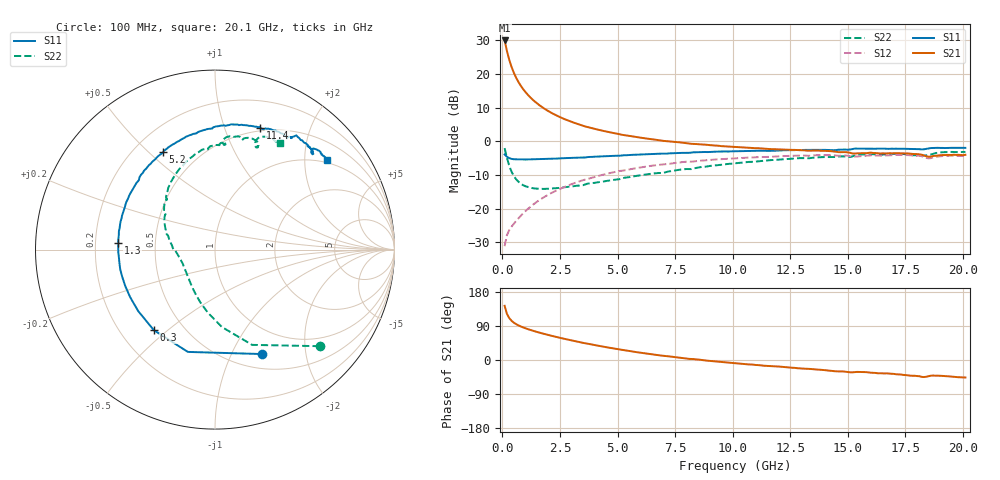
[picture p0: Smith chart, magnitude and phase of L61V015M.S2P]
!  Infineon Technologies AG
! BFR380L3 , PF131585-7, No.6, Th 09.10.01, soldered on pcb-board, measured with PP GSG850
!  Vce=1.0 V,  Ic=15.0 mA
! Common Emitter S-Parameters:  15. November 2001
#  GHz  S  MA  R  50
! f  S11  S21  S12  S22
! GHz  Mag  Ang  Mag  Ang  Mag  Ang  Mag  Ang
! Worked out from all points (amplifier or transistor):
!   201 points, 100 MHz to 20.1 GHz, reference 50 ohm
!   highest |S21| = 30.0 dB at 100 MHz (marker M1)
!   |S21| within 3 dB of that: start of sweep to 197.3 MHz
!   unconditionally stable (mu >= 1): 1.468 GHz to 4.926 GHz
!   at 3.4 GHz: K = 1.03, MAG = 7.3 dB, |S12| = -11.8 dB
!   at 10.1 GHz: K = 0.97, MSG = 1.7 dB, |S12| = -5.1 dB
!   at 20.1 GHz: K = 0.99, MSG = 0.1 dB, |S12| = -4.3 dB
!   S11 on the Smith chart (normalised r, x): 100 MHz: 0.67, -1.32; 300 MHz: 0.34, -0.45; 1.3 GHz: 0.30, +0.03; 5.2 GHz: 0.32, +0.56; 11.4 GHz: 0.47, +1.33; 20.1 GHz: 0.93, +2.56
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0.1  0.639 -65.6  31.62 142.9  0.02762 61.6  0.7934 -42.7
0.2  0.5897 -104.9  22.17 122.0  0.04024 52.2  0.5698 -68.7
0.3  0.5636 -127.2  16.36 110.8  0.04772 49.6  0.434 -84.8
0.4  0.5481 -141.4  12.81 103.6  0.05378 50.0  0.3545 -96.4
0.5  0.5419 -151.0  10.47 98.5  0.05958 51.7  0.3051 -105.5
0.6  0.5396 -158.0  8.824 94.7  0.06574 53.2  0.2728 -112.9
0.7  0.5387 -163.4  7.636 91.4  0.07169 54.7  0.2506 -119.4
0.8  0.5394 -168.1  6.721 88.5  0.0783 56.2  0.2347 -124.8
0.9  0.5378 -172.0  6.002 86.1  0.08483 57.2  0.2232 -129.6
1  0.5372 -175.5  5.43 83.8  0.09152 58.0  0.2153 -133.9
1.3  0.5404 176.2  4.222 77.7  0.1122 59.6  0.2017 -144.1
1.7  0.5446 167.4  3.272 70.7  0.1402 59.8  0.1968 -154.0
2.1  0.5516 159.8  2.687 64.5  0.1686 58.9  0.1985 -161.4
2.7  0.5615 149.8  2.14 55.8  0.2099 56.4  0.2077 -170.6
3.5  0.5738 138.2  1.707 45.3  0.2646 51.9  0.2226 -179.7
5.2  0.6167 118.0  1.25 26.6  0.3655 40.3  0.2796 162.7
6.8  0.6536 101.5  1.039 12.4  0.448 29.6  0.3384 145.2
10.1  0.7114 77.1  0.8238 -8.6  0.5591 8.4  0.472 118.0
11.4  0.7231 69.7  0.7752 -15.3  0.5856 0.3  0.5168 107.9
13.5  0.7463 60.0  0.7282 -24.3  0.6165 -11.5  0.5705 93.4
16.8  0.7736 47.7  0.6661 -35.9  0.619 -26.7  0.6474 74.1
20.1  0.7995 38.6  0.6303 -46.1  0.6125 -39.9  0.6954 58.9
